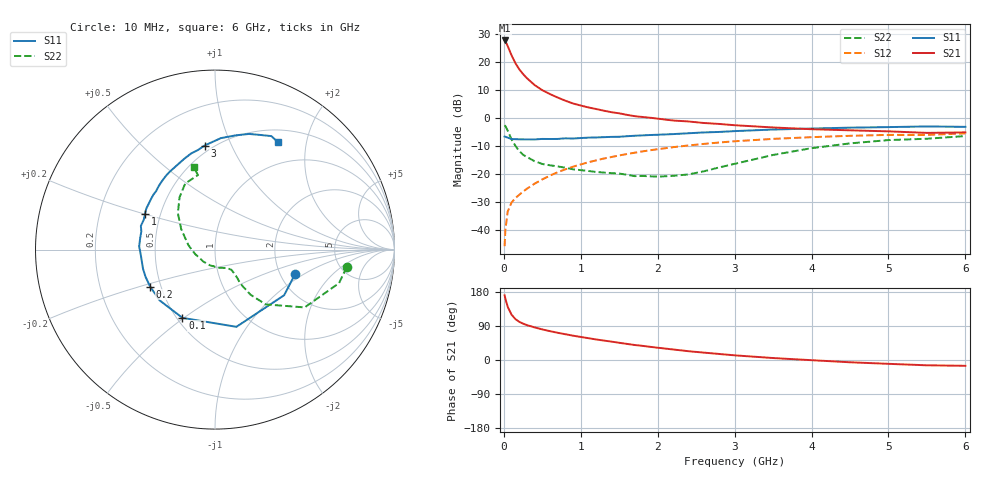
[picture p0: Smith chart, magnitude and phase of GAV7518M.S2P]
! Infineon Technologies  Discrete & RF Semiconductors
! BF775
! Si NPN RF Bipolar Junction Transistor in SOT23
! VCE = 0.75 V  IC = 18 mA
! Common Emitter S-Parameters:  May  1996
# GHz  S  MA  R  50
!  f  S11  S21  S12  S22
! GHz  MAG  ANG  MAG  ANG  MAG  ANG  MAG  ANG
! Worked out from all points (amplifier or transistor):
!   36 points, 10 MHz to 6 GHz, reference 50 ohm
!   highest |S21| = 27.6 dB at 10 MHz (marker M1)
!   |S21| within 3 dB of that: start of sweep to 65.49 MHz
!   unconditionally stable (mu >= 1): start of sweep to 16.31 MHz; 127.5 MHz to end of sweep
!   at 250 MHz: K = 1.39, MAG = 17.2 dB, |S12| = -26.2 dB
!   at 1.4 GHz: K = 1.62, MAG = 3.4 dB, |S12| = -13.9 dB
!   at 6 GHz: K = 1.16, MAG = -2.2 dB, |S12| = -5.5 dB
!   S11 on the Smith chart (normalised r, x): 10 MHz: 2.40, -0.84; 100 MHz: 0.53, -0.49; 200 MHz: 0.44, -0.22; 1 GHz: 0.41, +0.20; 3 GHz: 0.45, +0.80; 6 GHz: 0.67, +1.54
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0.01  0.4665 -17.1  24.01 170.7  0.0052 79.1  0.7399 -7.6
0.02  0.4615 -33.4  23.23 161.9  0.0102 73.3  0.716 -15.1
0.05  0.4465 -74.5  19.12 140.5  0.0214 62.4  0.5946 -32.8
0.1  0.4213 -115.5  13.07 119.6  0.0312 53.6  0.4155 -47.3
0.15  0.4186 -137.5  9.496 108.0  0.0373 54.2  0.3185 -51.8
0.2  0.4159 -150.2  7.361 100.8  0.0428 55.5  0.2571 -52.9
0.25  0.4157 -158.8  6.051 95.9  0.0487 57.3  0.2215 -52.8
0.3  0.415 -165.3  5.109 92.0  0.0548 59.6  0.2011 -51.9
0.4  0.4144 -175.8  3.855 86.0  0.0675 62.0  0.1697 -51.1
0.5  0.4229 177.6  3.122 80.7  0.0805 63.4  0.1514 -51.0
0.6  0.4218 171.4  2.66 76.1  0.094 64.0  0.1434 -51.2
0.7  0.4228 166.1  2.309 71.8  0.108 63.9  0.1369 -52.8
0.9  0.4303 157.0  1.809 64.2  0.1354 62.9  0.1216 -57.3
1  0.4386 152.8  1.663 60.8  0.1488 62.2  0.1176 -60.5
1.1  0.446 149.0  1.539 57.6  0.1624 61.3  0.1136 -64.7
1.7  0.4814 128.2  1.076 39.6  0.2403 53.6  0.092 -94.8
2.2  0.5156 114.2  0.9 27.8  0.3013 46.2  0.093 -134.0
3  0.5828 95.7  0.742 12.3  0.3843 33.4  0.1523 169.4
3.5  0.6219 87.0  0.677 5.2  0.4237 25.7  0.2192 149.0
4.5  0.6717 73.6  0.602 -6.0  0.4807 11.4  0.3522 124.1
5.5  0.7059 63.6  0.542 -14.0  0.4991 -1.7  0.4261 102.9
6  0.6938 59.6  0.553 -15.3  0.5311 -5.5  0.476 104.5
